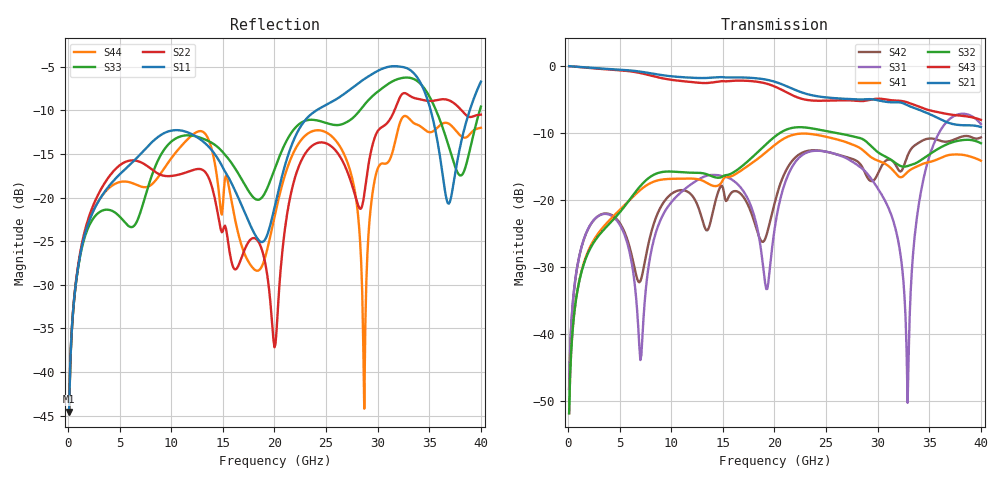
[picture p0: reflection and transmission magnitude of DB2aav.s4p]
! ADC12DJ2700AAV, ADC12DJ3200AAV, ADC08DJ3200AAV
! 144 pin AAV package
! Texas Instruments 4/21/2021
! Single-ended  S-parameters
! PORT#  PORT_NAME  NET_NAME
! PORT1:  DAxN.DIEBUMP DAxN
! PORT2:  DAxN.BGA  DAxN
! PORT3:  DAxP.DIEBUMP DAxP
! PORT4:  DAxP.BGA  DAxP
! Touchstone Ver. 1.0
! Number of ports is 4
# Hz	S	MA	R	50.000000
! SCATTERING PARAMETERS  :
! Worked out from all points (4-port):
!   400 points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, 100 MHz to 40 GHz, reference 50 ohm
!   strongest paths, dB at 100 MHz, 10.1 GHz, 20.1 GHz, 30.1 GHz, 40 GHz:
!     S21: 0.0, -1.5, -2.4, -5.1, -9.1
!     S43: 0.0, -2.1, -3.1, -4.9, -8.0
!     S32: -51.9, -15.8, -10.5, -13.0, -11.5
!     S41: -51.9, -16.9, -11.7, -14.2, -14.1
!     S31: -48.2, -20.2, -23.5, -18.5, -8.7
!     S42: -48.2, -19.0, -20.0, -15.8, -10.7
!   lowest |S11| = -44.5 dB at 100 MHz (marker M1), VSWR 1.01, Z = 50.3 + j0.532 ohm
!   |S11| at or under -10 dB: start of sweep to 24.05 GHz; 35.14 GHz to 38.92 GHz (3.776 GHz wide, 10.2 % of centre)
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1e8  0.005928 63.3  0.997 -1.9  0.003873 84.1  0.002542 -97.8
     0.997 -1.9  0.005946 62.2  0.002542 -97.8  0.003869 84.0
     0.003873 84.1  0.002542 -97.8  0.005807 64.1  0.9972 -1.8
     0.002542 -97.8  0.003869 84.0  0.9972 -1.8  0.005804 63.5
1.03e10  0.2437 -14.9  0.834 -171.4  0.102 66.5  0.1437 56.3
         0.834 -171.4  0.1339 -104.3  0.1622 66.4  0.1144 30.0
         0.102 66.5  0.1622 66.4  0.2161 11.5  0.7831 -163.2
         0.1437 56.3  0.1144 30.0  0.7831 -163.2  0.1774 -69.2
2.43e10  0.3229 -14.7  0.5916 -41.6  0.2326 22.6  0.3038 169.0
         0.5916 -41.6  0.2069 -79.8  0.3345 -174.4  0.2337 -52.4
         0.2326 22.6  0.3345 -174.4  0.2759 21.7  0.55 -12.0
         0.3038 169.0  0.2337 -52.4  0.55 -12.0  0.2435 -68.3
2.87e10  0.4786 -47.5  0.5638 -108.7  0.1659 -22.6  0.2302 77.2
         0.5638 -108.7  0.1043 -57.0  0.2797 96.9  0.164 -176.7
         0.1659 -22.6  0.2797 96.9  0.3402 1.9  0.5486 -74.3
         0.2302 77.2  0.164 -176.7  0.5486 -74.3  0.00617 -62.0
3.29e10  0.55 -105.5  0.5085 176.3  0.003044 -129.6  0.1615 28.5
         0.5085 176.3  0.3909 -96.9  0.179 44.0  0.2142 136.5
         0.003044 -129.6  0.179 44.0  0.4881 -52.9  0.5343 -146.0
         0.1615 28.5  0.2142 136.5  0.5343 -146.0  0.2896 -73.0
3.47e10  0.3833 -147.7  0.4484 145.6  0.1744 93.9  0.1891 -0.4
         0.4484 145.6  0.3599 -110.6  0.2105 24.1  0.2845 102.9
         0.1744 93.9  0.2105 24.1  0.4084 -90.0  0.4747 -175.1
         0.1891 -0.4  0.2845 102.9  0.4747 -175.1  0.2417 -87.1
4e10  0.4627 -26.7  0.3503 63.8  0.3686 -43.2  0.1961 -114.7
      0.3503 63.8  0.2992 -126.5  0.2649 -94.2  0.2927 62.7
      0.3686 -43.2  0.2649 -94.2  0.3328 53.5  0.3961 99.0
      0.1961 -114.7  0.2927 62.7  0.3961 99.0  0.2516 -90.1
